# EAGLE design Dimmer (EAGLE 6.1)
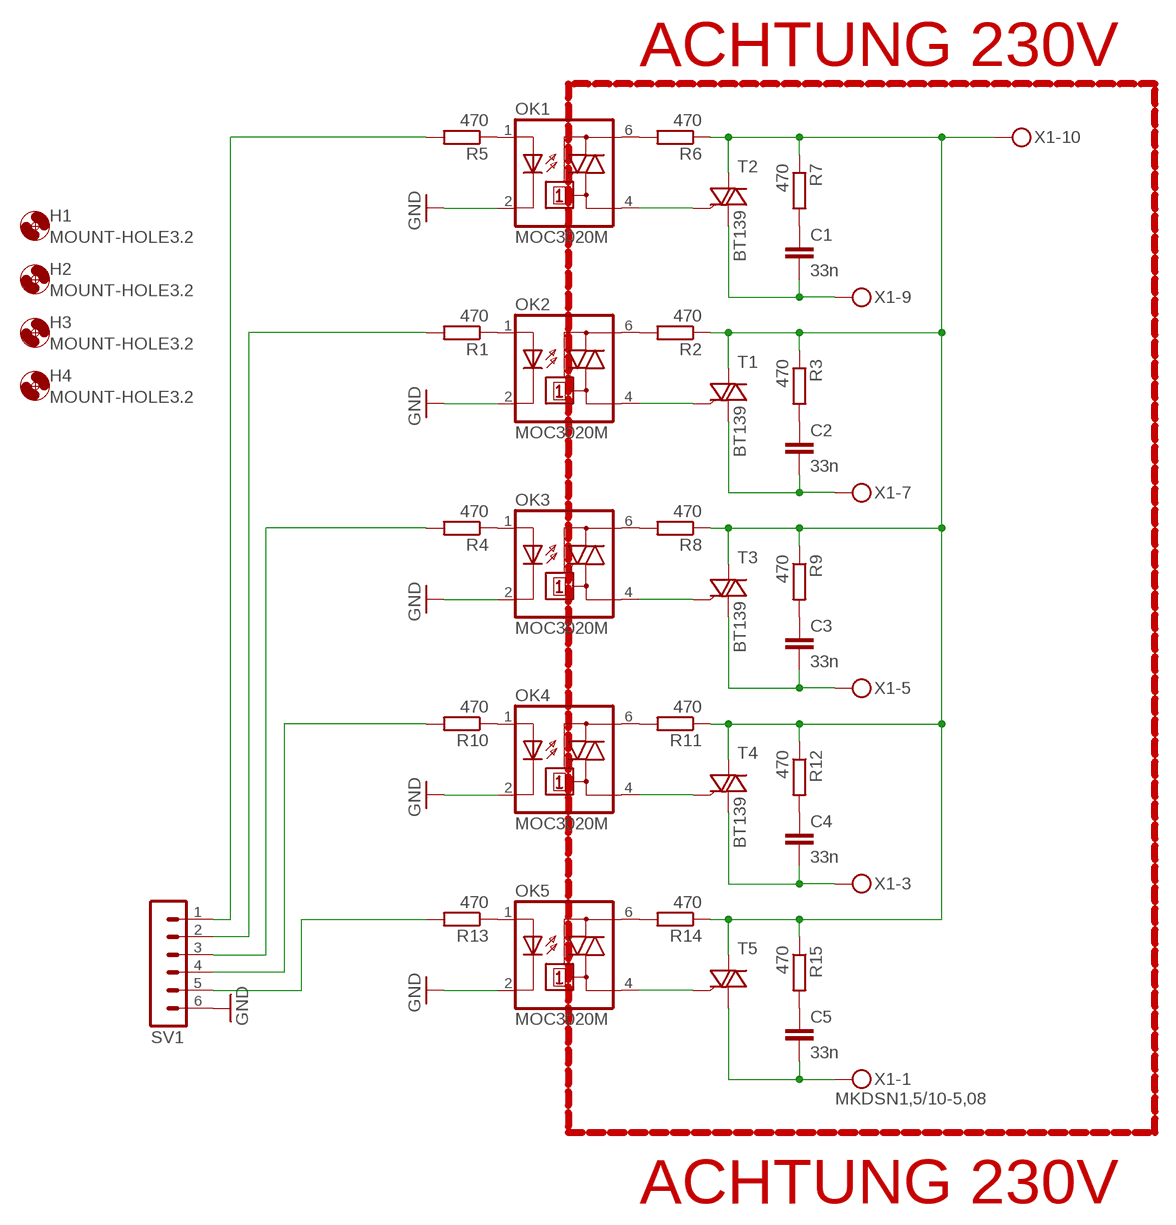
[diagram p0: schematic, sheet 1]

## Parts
C1  33n  C-EU075-052X106  [C075-052X106]
C2  33n  C-EU075-052X106  [C075-052X106]
C3  33n  C-EU075-052X106  [C075-052X106]
C4  33n  C-EU075-052X106  [C075-052X106]
C5  33n  C-EU075-052X106  [C075-052X106]
H1  MOUNT-HOLE3.2  [3,2]
H2  MOUNT-HOLE3.2  [3,2]
H3  MOUNT-HOLE3.2  [3,2]
H4  MOUNT-HOLE3.2  [3,2]
OK1  MOC3020M  [DIL06]
OK2  MOC3020M  [DIL06]
OK3  MOC3020M  [DIL06]
OK4  MOC3020M  [DIL06]
OK5  MOC3020M  [DIL06]
R1  470  R-EU_0204/7  [0204/7]
R2  470  R-EU_0204/7  [0204/7]
R3  470  R-EU_0204/7  [0204/7]
R4  470  R-EU_0204/7  [0204/7]
R5  470  R-EU_0204/7  [0204/7]
R6  470  R-EU_0204/7  [0204/7]
R7  470  R-EU_0204/7  [0204/7]
R8  470  R-EU_0204/7  [0204/7]
R9  470  R-EU_0204/7  [0204/7]
R10  470  R-EU_0204/7  [0204/7]
R11  470  R-EU_0204/7  [0204/7]
R12  470  R-EU_0204/7  [0204/7]
R13  470  R-EU_0204/7  [0204/7]
R14  470  R-EU_0204/7  [0204/7]
R15  470  R-EU_0204/7  [0204/7]
SV1  MA06-1  [MA06-1]
T1  BT138-V  [TO220BV]
T2  BT138-V  [TO220BV]
T3  BT138-V  [TO220BV]
T4  BT138-V  [TO220BV]
T5  BT138-V  [TO220BV]
X1  MKDSN1,5/10-5,08  [MKDSN1,5/10-5,08]

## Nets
GND: OK1.2(C) OK2.2(C) OK3.2(C) OK4.2(C) OK5.2(C) SV1.6
N$1: C5.2 T5.T1(A1) X1.1
N$2: OK2.1(A) R1.1
N$3: R4.2 SV1.3
N$4: OK2.6(A2) R2.2
N$5: C1.1 R7.2
N$6: R2.1 R3.1 R6.1 R7.1 R8.1 R9.1 R11.1 R12.1 R14.1 R15.1 T1.T2(A2) T2.T2(A2) T3.T2(A2) T4.T2(A2) T5.T2(A2) X1.10
N$7: C2.2 T1.T1(A1) X1.7
N$8: OK2.4(A1) T1.G
N$9: C2.1 R3.2
N$10: OK3.1(A) R4.1
N$11: R5.2 SV1.1
N$12: OK3.6(A2) R8.2
N$13: C3.1 R9.2
N$14: C4.1 R12.2
N$15: C3.2 T3.T1(A1) X1.5
N$16: OK3.4(A1) T3.G
N$17: R13.2 SV1.5
N$18: OK4.1(A) R10.1
N$19: R1.2 SV1.2
N$20: OK4.6(A2) R11.2
N$21: C5.1 R15.2
N$22: OK1.1(A) R5.1
N$24: C4.2 T4.T1(A1) X1.3
N$25: OK4.4(A1) T4.G
N$27: OK5.1(A) R13.1
N$30: OK1.4(A1) T2.G
N$31: OK1.6(A2) R6.2
N$34: C1.2 T2.T1(A1) X1.9
N$35: OK5.6(A2) R14.2
N$36: R10.2 SV1.4
N$39: OK5.4(A1) T5.G
Unconnected: X1.2 X1.4 X1.6 X1.8

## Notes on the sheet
- ACHTUNG 230V
- BT139
- BT139
- BT139
- BT139
- ACHTUNG 230V

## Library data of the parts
C1-C5 = rcl:C-EU: CAPACITOR, European symbol
H1-H4 = holes:MOUNT-HOLE: MOUNTING HOLE with drill center marker
OK1-OK5 = optocoupler:MOC30*M: RANDOM-PHASE OPTOISOLATORS TRIAC DRIVER OUTPUT Source: http://www.fairchildsemi.com MOC3020-M.pdf
R1-R15 = resistor:R-EU_: RESISTOR, European symbol
SV1 = con-lstb:MA06-1: PIN HEADER
T1-T5 = triac:BT138: TRIAC Source: http://www.semiconductors.philips.com BT138_SERIES_2.pdf
X1 = con-phoenix-508:MKDSN1,5/10-5,08: MKDSN 1,5/10-5,08 Printklemme Nennstrom: 13,5 A Nennspannung: 250 V Rastermaß: 5,08 mm Polzahl: 10 Anschlussart: Schraubanschluss Montage: Löten Anschlussrichtung Leiter/Platine: 0 ° Artikelnummer: 1729209 Source: http://eshop.phoenixcontact.com .. 1729209.pdf

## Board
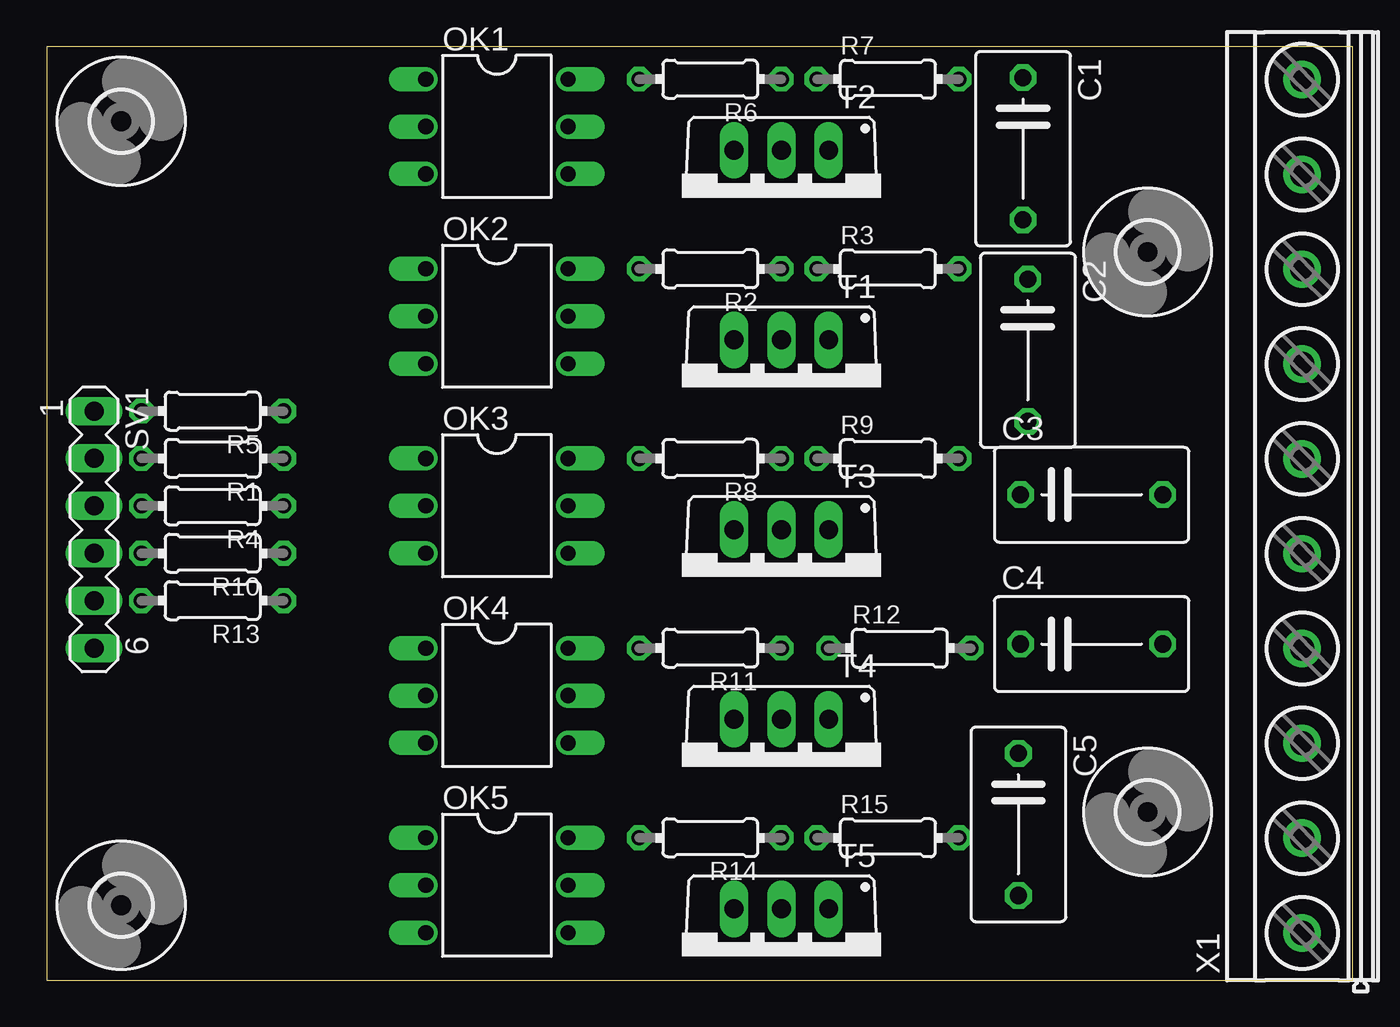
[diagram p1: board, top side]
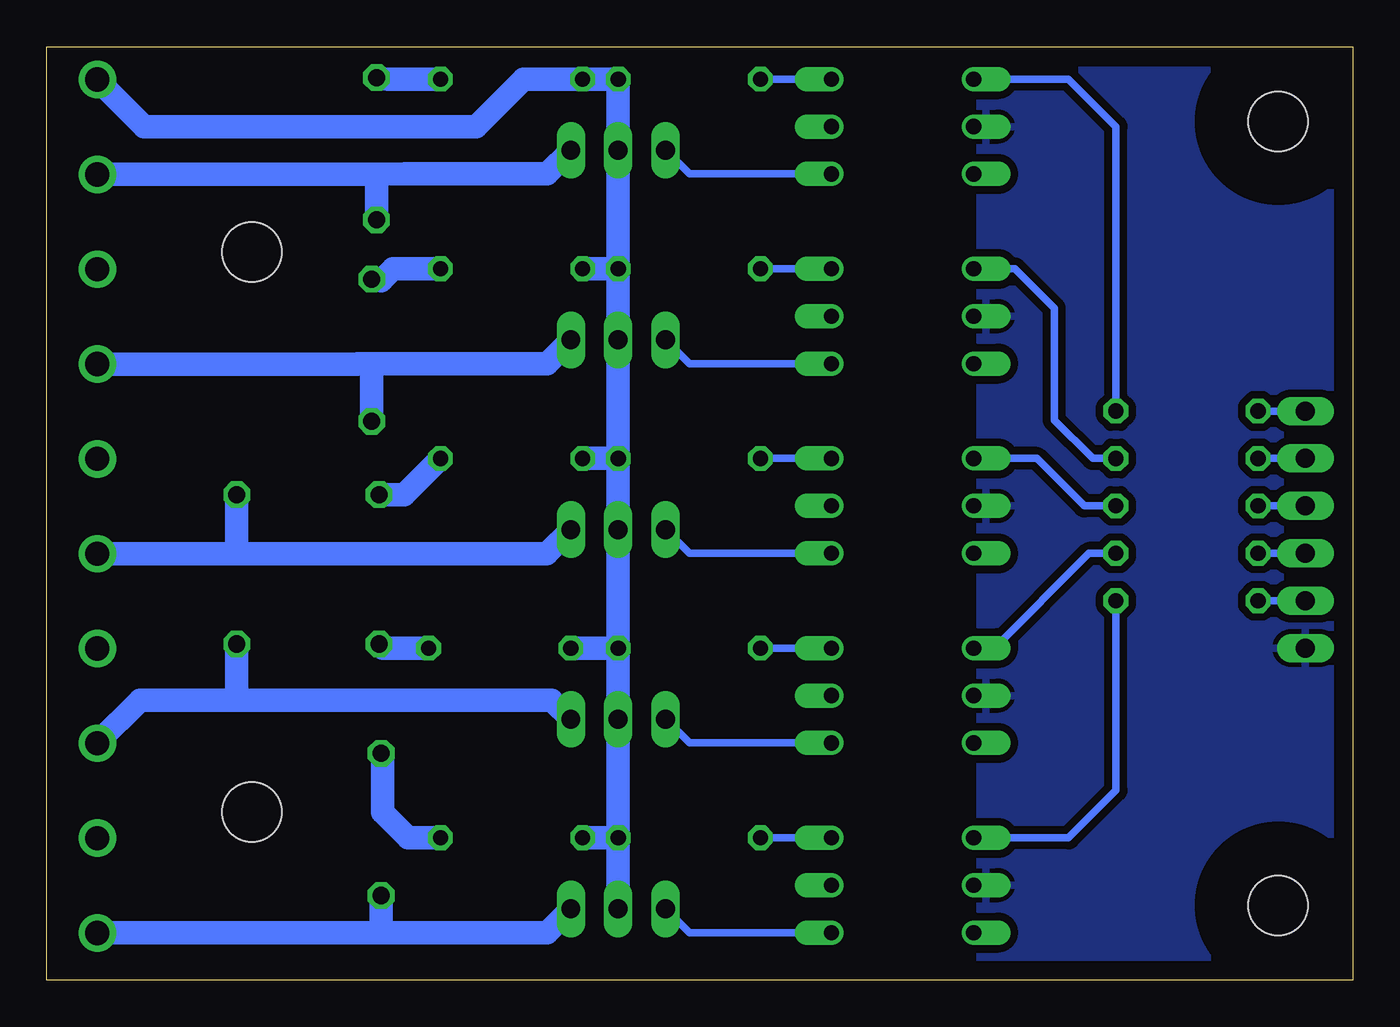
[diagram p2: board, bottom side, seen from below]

Size 70 x 50 mm. Coordinates in mm from the lower left corner, seen from the top.
Outline: 0,0 70,0 70,50 0,50 0,0
Copper layers (1*16): Top 0.035mm / dielectric 1.5mm / Bottom 0.035mm
Design rules: minimum track width 10mil, minimum drill 24mil, track to track 8mil, track to pad 8mil, pad to pad 8mil, via to via 8mil, smd to smd 8mil, copper to edge 40mil, drill to drill 8mil, minimum pad ring 10mil, minimum via ring 8mil, stop-mask expansion 4mil, vias tented up to drill 0mil, thermal gap 10mil

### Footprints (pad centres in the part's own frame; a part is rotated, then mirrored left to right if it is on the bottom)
C075-052X106 = drill 0.914 octagon: 1 -3.81,0; 2 3.81,0
3,2 = hole 3.2: 0,0
DIL06 = drill 0.813 offset: 1 -2.54,-3.81; 2 0,-3.81; 3 2.54,-3.81; 4 2.54,3.81; 5 0,3.81; 6 -2.54,3.81
0204/7 = drill 0.813 octagon: 1 -3.81,0; 2 3.81,0
MA06-1 = drill 1.016 long: 1 -6.35,0; 2 -3.81,0; 3 -1.27,0; 4 1.27,0; 5 3.81,0; 6 6.35,0
TO220BV = drill 1.016 long: G 2.54,-2.54; T1 -2.54,-2.54; T2 0,-2.54
MKDSN1,5/10-5,08 = drill 1.3 pad 2: 1 -22.881,0.025; 2 -17.801,0.025; 3 -12.721,0.025; 4 -7.641,0.025; 5 -2.561,0.025; 6 2.519,0.025; 7 7.599,0.025; 8 12.679,0.025; 9 17.759,0.025; 10 22.839,0.025

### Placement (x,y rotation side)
C1  52.33,44.53 270 top
C2  52.58,33.73 270 top
C3  56,26 0 top
C4  56,18 0 top
C5  52.08,8.34 270 top
H1  4,4 0 top
H2  4,46 0 top
H3  59,9 0 top
H4  59,39 0 top
OK1  24.13,45.72 270 top
OK2  24.13,35.56 270 top
OK3  24.13,25.4 270 top
OK4  24.13,15.24 270 top
OK5  24.13,5.08 270 top
R1  8.89,27.94 180 top
R2  35.56,38.1 180 top
R3  45.09,38.1 0 top
R4  8.89,25.4 180 top
R5  8.89,30.48 180 top
R6  35.56,48.26 180 top
R7  45.09,48.26 0 top
R8  35.56,27.94 180 top
R9  45.09,27.94 0 top
R10  8.89,22.86 180 top
R11  35.56,17.78 180 top
R12  45.72,17.78 0 top
R13  8.89,20.32 180 top
R14  35.56,7.62 180 top
R15  45.09,7.62 0 top
SV1  2.54,24.13 270 top
T1  39.37,31.75 180 top
T2  39.37,41.91 180 top
T3  39.37,21.59 180 top
T4  39.37,11.43 180 top
T5  39.37,1.27 180 top
X1  67.31,25.4 90 top

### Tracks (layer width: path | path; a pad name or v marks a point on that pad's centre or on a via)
GND
  pour Bottom (isolate 0.406): 1,49 1,1 20,1 20,49
N$1
  Bottom 1.27: X1.1 53.36,2.52 52.07,2.52 | T5.T1 43.18,2.54 43.2,2.52 52.07,2.52 | C5.2 52.08,2.52 52.07,2.52
N$2
  Bottom 0.406: R1.1 13.94,27.94 16,30 16,36 18.1,38.1 OK2.1
N$3
  Bottom 0.406: SV1.3 R4.2
N$4
  Bottom 0.406: OK2.6 R2.2
N$5
  Bottom 1.27: R7.2 51.44,48.26 51.69,48.26 C1.1
N$6
  Bottom 1.27: R11.1 T4.T2 R14.1 | R11.1 R12.1 | R8.1 T3.T2 R11.1 | R8.1 R9.1 | R2.1 T1.T2 R8.1 | R2.1 R3.1 | R14.1 R15.1 | T5.T2 R14.1 | X1.10 64.77,45.72 46.99,45.72 44.45,48.26 R7.1 R6.1 T2.T2 R2.1
N$7
  Bottom 1.27: X1.7 53.36,33 53.34,33.02 52,33.02 | T1.T1 43.18,33.02 52,33.02 | C2.2 52.58,32.97 52,33.02
N$8
  Bottom 0.406: OK2.4 35.56,33.02 T1.G
N$9
  Bottom 1.27: R3.2 51.44,38.1 52.07,37.47 51.99,37.55 C2.1
N$10
  Bottom 0.406: OK3.1 16.94,27.94 14.4,25.4 R4.1
N$11
  Bottom 0.406: SV1.1 R5.2
N$12
  Bottom 0.406: OK3.6 R8.2
N$13
  Bottom 1.27: C3.1 50.84,26 R9.2
N$14
  Bottom 1.27: R12.2 51.97,17.78 C4.1
N$15
  Bottom 1.27: 60,22.84 53.36,22.84 43.2,22.84 43.18,22.86 T3.T1 | 60,22.84 X1.5 | C3.2 59.81,23.03 60,22.84
N$16
  Bottom 0.406: OK3.4 35.56,22.86 T3.G
N$17
  Bottom 0.406: SV1.5 R13.2
N$18
  Bottom 0.406: R10.1 14.14,22.86 19.22,17.78 OK4.1
N$19
  Bottom 0.406: SV1.2 R1.2
N$20
  Bottom 0.406: OK4.6 R11.2
N$21
  Bottom 1.27: R15.2 50.62,7.62 52,9 52,12.07 C5.1
N$22
  Bottom 0.406: R5.1 12.7,45.72 15.24,48.26 OK1.1
N$24
  Bottom 1.27: X1.3 67.28,12.71 65,15 60,15 | 60,15 55.64,15 42.94,15 T4.T1 | C4.2 59.81,15.19 60,15
N$25
  Bottom 0.406: OK4.4 35.56,12.7 T4.G
N$27
  Bottom 0.406: R13.1 12.7,10.16 15.24,7.62 OK5.1
N$30
  Bottom 0.406: OK1.4 35.56,43.18 T2.G
N$31
  Bottom 0.406: OK1.6 R6.2
N$34
  Bottom 1.27: 52.73,43.16 X1.9 | T2.T1 43.18,43.18 50.8,43.2 52.73,43.16 | 52.73,43.16 52.33,43.16 C1.2
N$35
  Bottom 0.406: OK5.6 R14.2
N$36
  Bottom 0.406: SV1.4 R10.2
N$39
  Bottom 0.406: OK5.4 35.56,2.54 T5.G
